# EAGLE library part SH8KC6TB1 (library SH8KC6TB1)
60V Dual Nch+Nch, SOP8, Power MOSFET Source: Datasheet
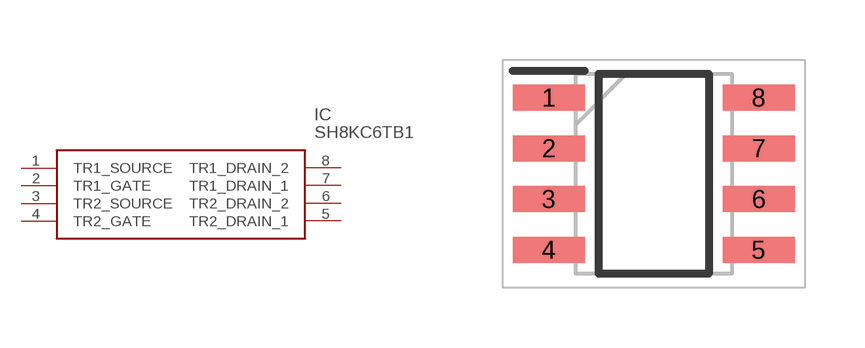
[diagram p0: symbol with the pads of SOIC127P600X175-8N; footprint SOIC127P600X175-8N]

Designator prefix IC

## SH8KC6TB1 (Description: 60V Dual Nch+Nch, SOP8, Power MOSFET; Height: 1.75mm; Manufacturer_Name: ROHM Semiconductor; Manufacturer_Part_Number: SH8KC6TB1; Mouser_Part_Number: 755-SH8KC6TB1; Mouser_Price-Stock: https://www.mouser.co.uk/ProductDetail/ROHM-Semiconductor/SH8KC6TB1?qs=QNEnbhJQKvZOtqarXY16MQ%3D%3D)  [SOIC127P600X175-8N]
1  TR1_SOURCE
2  TR1_GATE
3  TR2_SOURCE
4  TR2_GATE
5  TR2_DRAIN_1
6  TR2_DRAIN_2
7  TR1_DRAIN_1
8  TR1_DRAIN_2

## Footprint SOIC127P600X175-8N (pad centres in mm)
8 lead sop
smd 1.8 x 0.65: 1 -2.625,1.905; 2 -2.625,0.635; 3 -2.625,-0.635; 4 -2.625,-1.905; 5 2.625,-1.905; 6 2.625,-0.635; 7 2.625,0.635; 8 2.625,1.905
